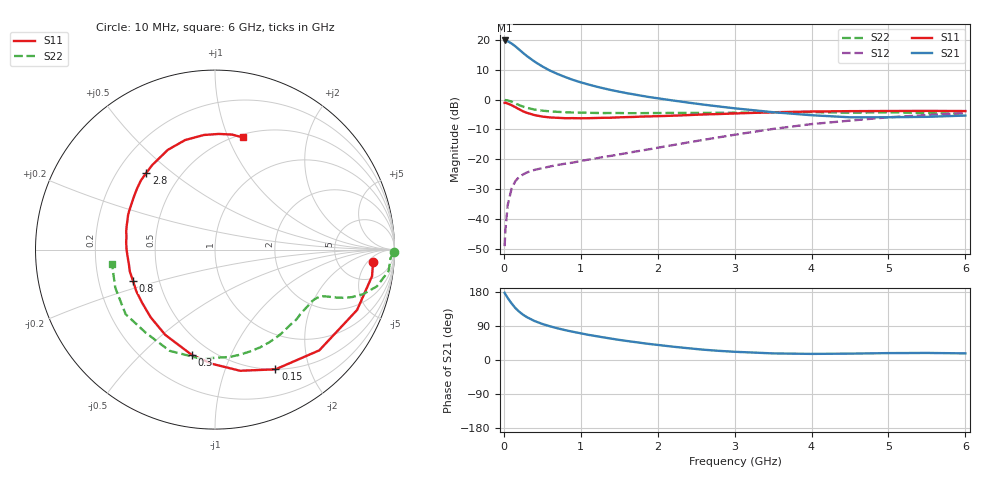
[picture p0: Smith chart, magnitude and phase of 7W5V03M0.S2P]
! Infineon Technologies  Discrete & RF Semiconductors
! BFS17W
! Si NPN RF Bipolar Junction Transistor in SOT323
! VCE = 5 V  IC = 3 mA
! Common Emitter S-Parameters:  August  1999
# GHz  S  MA  R  50
!  f  S11  S21  S12  S22
! GHz  MAG  ANG  MAG  ANG  MAG  ANG  MAG  ANG
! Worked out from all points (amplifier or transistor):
!   36 points, 10 MHz to 6 GHz, reference 50 ohm
!   highest |S21| = 19.8 dB at 10 MHz (marker M1)
!   |S21| within 3 dB of that: start of sweep to 197 MHz
!   unconditionally stable (mu >= 1): 725.3 MHz to 2.813 GHz; 4.322 GHz to end of sweep
!   at 250 MHz: K = 0.44, MSG = 20.4 dB, |S12| = -25.1 dB
!   at 1.4 GHz: K = 1.26, MAG = 7.9 dB, |S12| = -18.8 dB
!   at 6 GHz: K = 1.08, MAG = -2.1 dB, |S12| = -4.6 dB
!   S11 on the Smith chart (normalised r, x): 10 MHz: 11, -7; 150 MHz: 0.50, -1.51; 300 MHz: 0.39, -0.73; 800 MHz: 0.35, -0.16; 2.8 GHz: 0.32, +0.41; 6 GHz: 0.53, +1.13
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0.01  0.8837 -4.6  9.818 177.3  0.0035 83.6  0.9982 -0.9
0.02  0.8874 -9.6  9.773 173.5  0.0065 86.8  0.9789 -2.8
0.05  0.8602 -23.0  9.535 163.7  0.017 78.9  0.9747 -7.0
0.1  0.808 -44.0  8.741 149.5  0.0321 67.9  0.9249 -12.8
0.15  0.7474 -63.2  7.827 137.0  0.0432 59.2  0.8626 -16.7
0.2  0.6894 -78.3  6.898 127.4  0.0508 54.2  0.8086 -19.1
0.25  0.6372 -91.2  6.065 119.5  0.0557 49.6  0.763 -20.6
0.3  0.6011 -102.4  5.379 113.0  0.0603 47.6  0.7296 -21.5
0.4  0.5499 -120.3  4.336 102.8  0.0665 45.1  0.6815 -22.6
0.5  0.5203 -133.5  3.606 95.2  0.0711 45.0  0.6542 -23.4
0.6  0.5029 -143.7  3.068 88.9  0.0758 45.6  0.6359 -24.5
0.8  0.4889 -159.3  2.387 78.7  0.0845 48.7  0.6149 -27.4
0.9  0.4899 -165.6  2.142 74.4  0.0883 50.0  0.6084 -29.1
1.1  0.489 -176.1  1.793 66.4  0.0988 53.5  0.602 -32.9
1.3  0.4966 175.3  1.544 59.5  0.1097 56.4  0.5961 -37.4
1.6  0.5102 164.5  1.283 50.2  0.1272 60.4  0.5934 -44.3
2.2  0.5383 147.4  0.967 35.1  0.1733 66.0  0.5985 -59.9
2.8  0.574 131.7  0.767 24.1  0.234 67.0  0.6019 -76.9
3.5  0.6148 115.3  0.616 17.4  0.323 63.7  0.6135 -97.5
4.5  0.6416 95.5  0.506 16.8  0.4453 51.9  0.6028 -129.8
5.5  0.6479 81.5  0.515 18.6  0.5509 38.9  0.595 -159.0
6  0.6437 76.2  0.541 17.5  0.5919 32.5  0.5795 -172.0
